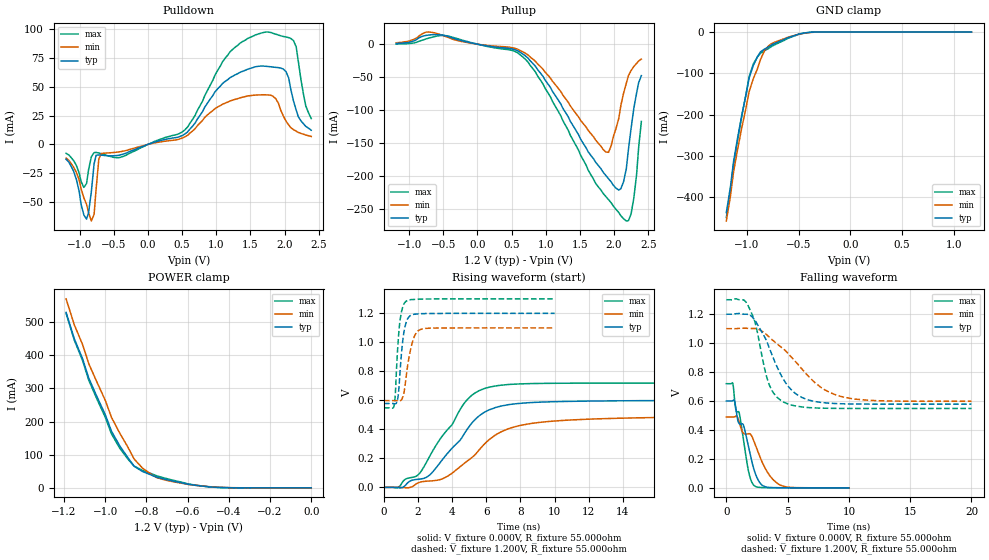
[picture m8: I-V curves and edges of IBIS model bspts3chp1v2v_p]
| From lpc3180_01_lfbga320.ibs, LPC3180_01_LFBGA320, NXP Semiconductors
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| |   Rev 0.20 IBIS Model Design Automation Generation   |
| |   N O N - S I L I C O N   C O R R E L A T E D   |
| |   This IBIS [Model] is pre-Beta tactical support   |
| |  Note: this IBIS [Model] contains clamp curves generated   |
| |   through simulation which should not be relied upon   |
| bspts3chp1v2v
|   Bidirectional Pad 1v2
|   3state Output
|   Plain Input
|   3ns Slew Rate control
|   CMOS
|   Programmable between
|   - (p1=0, p2=1) plain input
|   - (p1=0, p2=0) with Pull Up
|   - (p1=1, p2=1) with Pull Down
|   - (p1=1, p2=0) with Repeater
|   Characterized at Core 1.2V and I/O 1.2V
| Plain input Mode (p1=0, p2=1)
[Model]   bspts3chp1v2v_p | of bspts3chp1v2v
Model_type   I/O
Polarity   Non-Inverting
Enable   Active-Low
|  Reciever Thresholds
Vinl   = 0.36V
Vinh   = 0.84V
| AC Test Load Conditions
Vref   = 0
Cref   = 1.2e-11
Rref   = 1000000000
Vmeas   = 0.6
| [Process Range]   typical   min   max
| C_comp edge width   400.000ps   400.000ps   400.000ps
| C_comp Tstrobe   40.000fs   40.000fs   40.000fs
C_comp   2.971pF   2.766pF   3.250pF
[Temperature Range]   25   105   -20
[Voltage Range]   1.20V   1.10V   1.30V
[GND Clamp Reference]   0.00V   0.00V   0.00V
[Pulldown Reference]   0.00V   0.00V   0.00V
[POWER Clamp Reference]   1.20V   1.10V   1.30V
[Pullup Reference]   1.20V   1.10V   1.30V
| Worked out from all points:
|   slope of the pulldown table from 0 to 0.18 V, typ, clamps not added: 55.1 ohm
|   slope of the pullup table from 0 to 0.18 V, typ, clamps not added: 53.4 ohm
|   GND clamp passes 1 mA (typ) near -0.40 V on its own axis
|   POWER clamp passes 1 mA (typ) near -0.44 V on its own axis
|   rising waveform, V_fixture 0.000V, R_fixture 55.000ohm: 20-80 % time 2.49ns typ, 3ns min, 2.32ns max; typ from 0 V to 0.6 V
|   falling waveform, V_fixture 0.000V, R_fixture 55.000ohm: 20-80 % time 1.38ns typ, 2.14ns min, 1.03ns max; typ from 0.601 V to 0 V
|   rising waveform, V_fixture 1.200V, R_fixture 55.000ohm: 20-80 % time 290ps typ, 434ps min, 251ps max; typ from 0.578 V to 1.2 V
|   falling waveform, V_fixture 1.200V, R_fixture 55.000ohm: 20-80 % time 2.13ns typ, 3.58ns min, 1.25ns max; typ from 1.2 V to 0.578 V
[GND Clamp]
| ref voltage   0.00V   0.00V   0.00V
|   Voltage   I(typ)   I(min)   I(max)
-1.2V     -437mA     -457.3mA   -448.8mA
-1.16V    -374mA     -396.6mA   -383.9mA
-1.13V    -313.1mA   -338.2mA   -320.8mA
-1.05V    -200.5mA   -230.7mA   -202.9mA
-980mV    -111.6mA   -144.4mA   -108mA
-940mV    -81.36mA   -113.4mA   -77.52mA
-870mV    -48.1mA    -66.67mA   -51.38mA
-830mV    -41.09mA   -44.62mA   -45.09mA
-790mV    -35.71mA   -33.02mA   -39.59mA
-570mV    -10.68mA   -10.1mA    -11.93mA
-390mV    -608.9uA   -1.074mA   -502.3uA
1.17V     1.021nA    183.7nA    430.8pA
[Power Clamp]   | Vtable = Vcc - Vpad
| ref voltage   1.20V   1.10V   1.30V
|   Voltage   I(typ)   I(min)   I(max)
-1.19V    529.3mA    570.1mA    526.5mA
-1.15V    449.5mA    491.7mA    445.3mA
-1.11V    389.5mA    432.5mA    384.2mA
-1.08V    331.1mA    374.7mA    324.8mA
-1V       221.2mA    264.5mA    213.3mA
-970mV    171.3mA    213.2mA    163.4mA
-890mV    91.01mA    122.9mA    86.95mA
-860mV    65.35mA    87.21mA    65.73mA
-820mV    49.49mA    60.15mA    53.03mA
-750mV    32.06mA    30.85mA    36.23mA
-560mV    7.514mA    7.557mA    8.063mA
0V        1.855nA    42.78nA    728.2pA
[Pulldown]
| ref voltage   0.00V   0.00V   0.00V
|   Voltage   I(typ)   I(min)   I(max)
-1.2V     -12.9mA    -11.81mA   -7.731mA
-900mV    -64.77mA   -51.94mA   -33.89mA
-830mV    -41mA      -66.41mA   -10.78mA
-760mV    -9.4mA     -38.72mA   -6.922mA
-720mV    -9.108mA   -12.34mA   -7.471mA
-680mV    -9.342mA   -7.831mA   -8.122mA
500mV     7.667mA    5.475mA    10.77mA
1.2V      57.8mA     37.61mA    80.16mA
1.72V     67.75mA    42.98mA    97.43mA
2.02V     63.12mA    20.22mA    93.1mA
2.13V     37.64mA    12.84mA    90mA
2.39V     12.34mA    6.89mA     22.38mA
[Pullup]   | Vtable = Vcc - Vpad
| ref voltage   1.20V   1.10V   1.30V
|   Voltage   I(typ)   I(min)   I(max)
-1.19V    982.9uA    2.112mA    262.9uA
-710mV    13.91mA    18.44mA    9.271mA
-450mV    12.25mA    11.02mA    12.78mA
590mV     -9.985mA   -7.698mA   -13.1mA
960mV     -48.84mA   -37.98mA   -60.41mA
1.88V     -199.3mA   -163.7mA   -231.3mA
1.96V     -209.3mA   -153.4mA   -241mA
2.07V     -221.5mA   -112.2mA   -255.7mA
2.18V     -188.7mA   -59.17mA   -268.4mA
2.25V     -127.4mA   -39.92mA   -257.5mA
2.33V     -74.26mA   -29.16mA   -198.1mA
2.4V      -47.75mA   -22.65mA   -117.4mA
[Ramp]
R_load   = 55.000ohm
|   dV/dt(typ)   dV/dt(min)   dV/dt(max)
dV/dt_r   338.121mV/2.450ns   259.420mV/2.715ns   412.951mV/2.315ns
dV/dt_f   356.465mV/2.200ns   272.411mV/3.340ns   434.042mV/1.325ns
[Rising Waveform]  | cubic spline decimation from 4001 points
V_fixture   = 0.000V
R_fixture   = 55.000ohm
|   Time   V(typ)   V(min)   V(max)
0s        163.2nV    2.488uV    162.3nV
755ps     -1.211mV   314.8uV    -2.714mV
1.945ns   55.13mV    27.44mV    80.98mV
2.57ns    75.24mV    43.12mV    190.4mV
3.51ns    203.8mV    63.29mV    368mV
4.8ns     387mV      174.2mV    594.3mV
6.01ns    525.9mV    313.1mV    685.9mV
7.275ns   569.8mV    403.6mV    709.1mV
9.245ns   588.1mV    449.7mV    716.9mV
20ns      599.7mV    486.4mV    719.6mV
[Falling Waveform]  | cubic spline decimation from 2001 points
V_fixture   = 0.000V
R_fixture   = 55.000ohm
|   Time   V(typ)   V(min)   V(max)
0s        600.6mV    489.7mV    719.8mV
525ps     602.1mV    489.7mV    722.3mV
755ps     562.9mV    494.5mV    549.4mV
1.055ns   443mV      452.1mV    516.5mV
1.4ns     432.4mV    377.7mV    331.9mV
1.815ns   283.1mV    374.1mV    113.1mV
2.29ns    117.7mV    313.6mV    13.93mV
2.96ns    15.87mV    171mV      1.953mV
4.305ns   950uV      23.38mV    337.8uV
10ns      7.631uV    93.34uV    1.442uV
[Rising Waveform]  | cubic spline decimation from 2001 points
V_fixture   = 1.200V
V_fixture_min = 1.100V
V_fixture_max = 1.300V
R_fixture   = 55.000ohm
|   Time   V(typ)   V(min)   V(max)
0s        578.5mV    598.3mV    548.6mV
600ps     576.9mV    598.3mV    567.3mV
670ps     576.2mV    598.3mV    651mV
800ps     607.2mV    596.8mV    950.1mV
925ps     765mV      596.2mV    1.134V
1.12ns    1.029V     628.2mV    1.251V
1.315ns   1.142V     775.8mV    1.285V
1.7ns     1.192V     1.014V     1.295V
2.165ns   1.198V     1.09V      1.298V
10ns      1.2V       1.1V       1.3V
[Falling Waveform]  | cubic spline decimation from 4001 points
V_fixture   = 1.200V
V_fixture_min = 1.100V
V_fixture_max = 1.300V
R_fixture   = 55.000ohm
|   Time   V(typ)   V(min)   V(max)
0s        1.2V       1.1V       1.3V
1.4ns     1.2V       1.103V     1.299V
1.77ns    1.199V     1.102V     1.26V
2.335ns   1.157V     1.101V     1.146V
3.495ns   969.5mV    1.042V     713.3mV
4.85ns    724.5mV    945.1mV    585.9mV
6.45ns    614.5mV    794mV      556.6mV
7.735ns   590.2mV    693.4mV    550.8mV
9.36ns    581.2mV    631.2mV    548.9mV
20ns      578.5mV    598.3mV    548.6mV
